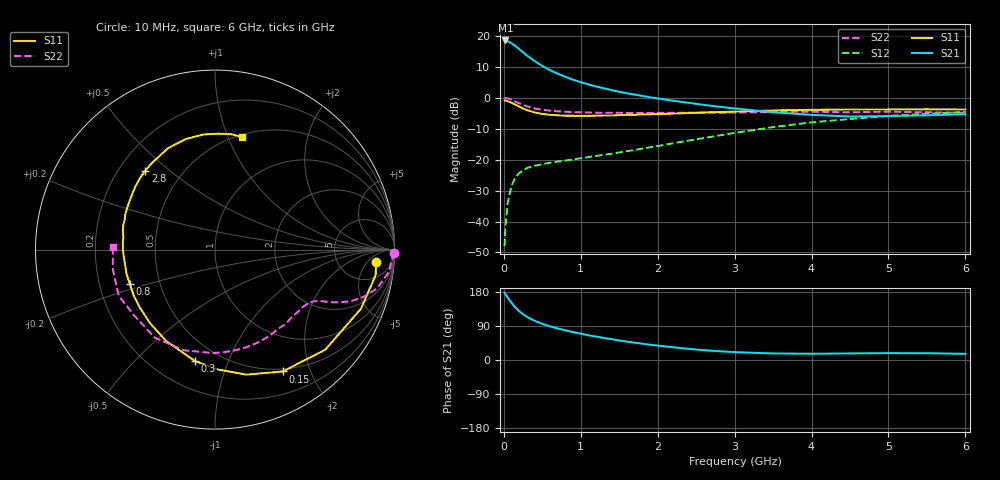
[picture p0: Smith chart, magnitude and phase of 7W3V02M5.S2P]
! Infineon Technologies  Discrete & RF Semiconductors
! BFS17W
! Si NPN RF Bipolar Junction Transistor in SOT323
! VCE = 3 V  IC = 2.5 mA
! Common Emitter S-Parameters:  August  1999
# GHz  S  MA  R  50
!  f  S11  S21  S12  S22
! GHz  MAG  ANG  MAG  ANG  MAG  ANG  MAG  ANG
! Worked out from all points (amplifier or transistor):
!   36 points, 10 MHz to 6 GHz, reference 50 ohm
!   highest |S21| = 18.5 dB at 20 MHz (marker M1)
!   |S21| within 3 dB of that: start of sweep to 209.5 MHz
!   unconditionally stable (mu >= 1): 751.6 MHz to 3.426 GHz; 3.662 GHz to end of sweep
!   at 250 MHz: K = 0.41, MSG = 19.1 dB, |S12| = -23.5 dB
!   at 1.4 GHz: K = 1.31, MAG = 6.9 dB, |S12| = -18.1 dB
!   at 6 GHz: K = 1.10, MAG = -2.2 dB, |S12| = -4.6 dB
!   S11 on the Smith chart (normalised r, x): 10 MHz: 13, -9; 150 MHz: 0.47, -1.60; 300 MHz: 0.37, -0.77; 800 MHz: 0.33, -0.17; 2.8 GHz: 0.31, +0.41; 6 GHz: 0.52, +1.12
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0.01  0.8991 -4.3  8.369 177.5  0.004 85.9  0.9983 -1.0
0.02  0.9064 -9.0  8.407 173.8  0.008 88.1  0.9886 -3.0
0.05  0.8777 -22.0  8.172 164.5  0.02 79.0  0.977 -7.3
0.1  0.8296 -42.2  7.554 150.8  0.0382 67.8  0.9297 -13.4
0.15  0.777 -60.9  6.827 138.5  0.0514 59.7  0.8665 -17.8
0.2  0.7183 -75.9  6.091 128.7  0.0607 53.8  0.8114 -20.7
0.25  0.6677 -88.8  5.39 120.7  0.0669 48.4  0.7621 -22.6
0.3  0.6314 -100.1  4.805 114.1  0.073 46.1  0.7264 -23.9
0.4  0.5772 -118.2  3.903 103.4  0.0796 42.2  0.6705 -25.5
0.5  0.5468 -131.5  3.254 95.5  0.0843 41.3  0.6399 -26.6
0.6  0.5288 -142.3  2.786 88.8  0.0889 41.3  0.6178 -27.9
0.8  0.5117 -158.2  2.171 78.2  0.0964 43.3  0.593 -31.2
0.9  0.5114 -164.6  1.954 73.6  0.1006 44.8  0.5849 -33.0
1.1  0.5097 -175.4  1.639 65.2  0.1098 47.9  0.5767 -37.3
1.3  0.5148 175.6  1.419 58.1  0.1197 51.0  0.5696 -42.2
1.6  0.5294 164.7  1.178 48.5  0.1365 55.4  0.5661 -49.8
2.2  0.5533 147.2  0.894 33.5  0.1838 61.5  0.5706 -66.9
2.8  0.5867 131.5  0.714 23.1  0.2457 62.8  0.5737 -85.2
3.5  0.6224 115.1  0.582 17.3  0.3353 59.3  0.5872 -107.1
4.5  0.6448 95.7  0.497 17.3  0.4525 47.5  0.5807 -140.2
5.5  0.6494 81.9  0.519 17.9  0.5504 35.0  0.5801 -168.8
6  0.6456 76.6  0.542 16.3  0.5884 28.9  0.5692 178.6
